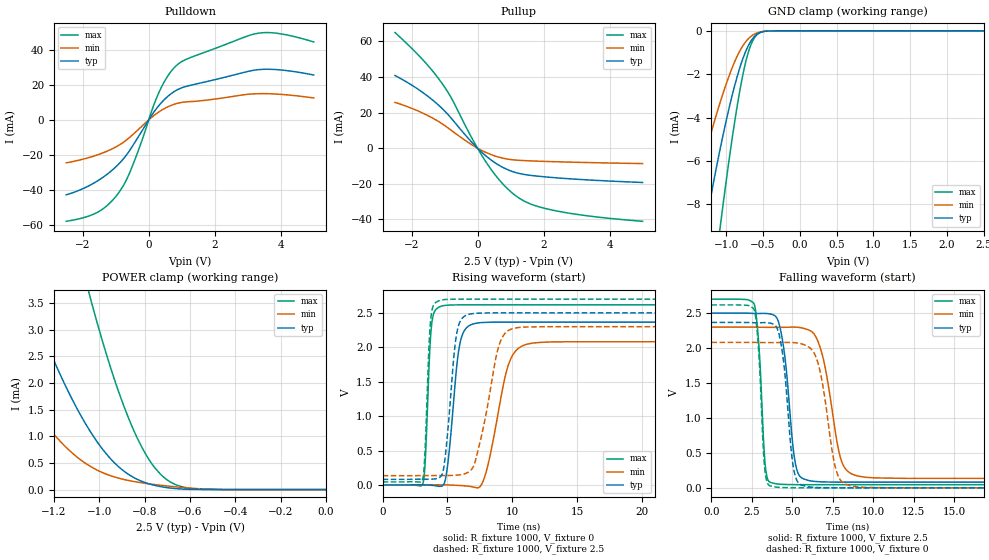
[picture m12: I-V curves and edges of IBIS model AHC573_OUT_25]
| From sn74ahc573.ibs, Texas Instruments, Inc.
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[Model]   AHC573_OUT_25
Model_type  3-state
Enable   Active-Low
Vref =   0.0
Rref =   1000
Cref =   50p
Vmeas =   1.25
| variable   typ   min   max
C_comp   2.25pF   1.96pF   2.41pF
| C_pullup   3.29pF   2.06pF   4.03pF
| C_pulldown   2.98pF   2.14pF   3.95pF
| C_tri-state   2.25pF   1.96pF   2.41pF
[Temperature Range]   40   100   -40
| Ambient temperature   25   85   -40
[Voltage range]   2.5   2.3   2.7
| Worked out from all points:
|   slope of the pulldown table from 0 to 0.375 V, typ, clamps not added: 38.9 ohm
|   slope of the pullup table from 0 to 0.375 V, typ, clamps not added: 61.3 ohm
|   GND clamp passes 1 mA (typ) near -0.74 V on its own axis
|   POWER clamp passes 1 mA (typ) near -1.03 V on its own axis
|   rising waveform, R_fixture 1000, V_fixture 0: 20-80 % time 696ps typ, 1.3ns min, 346ps max; typ from 0 V to 2.37 V
|   falling waveform, R_fixture 1000, V_fixture 2.5: 20-80 % time 597ps typ, 941ps min, 357ps max; typ from 2.5 V to 0.082 V
|   rising waveform, R_fixture 1000, V_fixture 2.5: 20-80 % time 663ps typ, 1.32ns min, 329ps max; typ from 0.082 V to 2.5 V
|   falling waveform, R_fixture 1000, V_fixture 0: 20-80 % time 548ps typ, 827ps min, 337ps max; typ from 2.37 V to 0 V
[GND Clamp]
| AHC573_OUT_25
|   Voltage   I(typ)   I(min)   I(max)
-2.5V     -38.12mA   -24.73mA   -54.32mA
-1.525V   -13.97mA   -8.89mA    -22.06mA
-1.285V   -9.079mA   -5.688mA   -14.78mA
-1.255V   -8.511mA   -5.315mA   -13.91mA
-1.085V   -5.504mA   -3.34mA    -9.154mA
-1.06V    -5.095mA   -3.072mA   -8.49mA
-940mV    -3.279mA   -1.897mA   -5.474mA
-805mV    -1.608mA   -872.9uA   -2.591mA
-710mV    -764.9uA   -407.8uA   -1.124mA
-610mV    -244uA     -144.1uA   -295.3uA
-415mV    -8.6uA     -6.443uA   -5.43uA
2.5V      4.776nA    2.156nA    12.02nA
[POWER Clamp]
| AHC573_OUT_25
|   Voltage   I(typ)   I(min)   I(max)
-2.5V     24.44mA    14.42mA    44.71mA
-1.57V    6.941mA    3.585mA    15.12mA
-1.315V   3.634mA    1.685mA    8.895mA
-1.185V   2.279mA    965.9uA    6.184mA
-1.06V    1.233mA    491.7uA    3.931mA
-1.035V   1.06mA     424.9uA    3.527mA
-935mV    511.3uA    239.6uA    2.092mA
-845mV    219.7uA    150.4uA    1.083mA
-780mV    107uA      108.3uA    559.4uA
-715mV    45.8uA     74.66uA    229.8uA
-585mV    3.146uA    22.88uA    17.46uA
-31.15fV  4.776nA    1.311nA    18.11nA
[Pulldown]
| AHC573_OUT_25
|   Voltage   I(typ)   I(min)   I(max)
-2.5V     -42.7mA    -24.49mA   -57.81mA
-1.54V    -34.65mA   -19.85mA   -52.55mA
-1.21V    -30.24mA   -17.4mA    -47.97mA
-895mV    -24.87mA   -14.36mA   -41.15mA
-495mV    -15.05mA   -8.58mA    -26.34mA
130mV     3.762mA    2.089mA    7.297mA
335mV     8.782mA    4.878mA    16.71mA
630mV     14.23mA    7.881mA    26.48mA
930mV     17.74mA    9.73mA     32.38mA
3.295V    28.59mA    14.93mA    49.33mA
3.97V     28.53mA    14.6mA     49.16mA
5V        25.59mA    12.52mA    44.44mA
[Pullup]
| AHC573_OUT_25
|   Voltage   I(typ)   I(min)   I(max)
-2.5V     40.85mA    25.73mA    64.98mA
-1.72V    32.11mA    20.24mA    50.94mA
-1.15V    23.68mA    14.65mA    38.34mA
-800mV    16.93mA    10.1mA     28.45mA
-175mV    3.382mA    1.944mA    5.825mA
250mV     -4.262mA   -2.344mA   -7.567mA
695mV     -10.06mA   -5.252mA   -18.61mA
1.135V    -13.57mA   -6.625mA   -26.4mA
1.61V     -15.26mA   -7.124mA   -31.38mA
2.33V     -16.56mA   -7.586mA   -35.02mA
3.45V     -17.93mA   -8.108mA   -38.28mA
5V        -19.26mA   -8.64mA    -41.08mA
[Ramp]
| AHC573_OUT_25
| variable   typ   min   max
dV/dt_r   1.43/7.06E-10   1.27/1.32E-09   1.58/3.57E-10
dV/dt_f   1.45/5.98E-10   1.30/9.44E-10   1.59/3.63E-10
R_load = 1000
[Rising Waveform]
| AHC573_OUT_25
R_fixture =   1000
C_fixture =   0
L_fixture =   0
V_fixture =   0
V_fixture_min = 0
V_fixture_max = 0
|   Time   V(typ)   V(min)   V(max)
0s        697.4pV    1.232nV    360.5pV
3.115ns   3.239mV    2.463mV    25.92mV
3.775ns   -4.622mV   3.276mV    2.315V
4.545ns   -18.6mV    2.071mV    2.599V
5.945ns   2.034V     -6.937mV   2.617V
7.015ns   2.341V     -29.59mV   2.617V
7.97ns    2.363V     174.8mV    2.617V
9.78ns    2.366V     1.783V     2.617V
11.16ns   2.366V     2.046V     2.617V
50ns      2.366V     2.081V     2.617V
[Falling Waveform]
| AHC573_OUT_25
R_fixture =   1000
C_fixture =   0
L_fixture =   0
V_fixture =   2.5
V_fixture_min = 2.3
V_fixture_max = 2.7
|   Time   V(typ)   V(min)   V(max)
0s        2.5V       2.3V       2.7V
2.645ns   2.496V     2.3V       2.63V
3.345ns   2.495V     2.297V     282.1mV
3.88ns    2.469V     2.296V     63.5mV
4.465ns   2.002V     2.297V     49.34mV
5.205ns   329mV      2.299V     45.99mV
6ns       105.4mV    2.26V      45.24mV
8.03ns    82.2mV     389.7mV    45.04mV
9.115ns   81.75mV    166mV      45.03mV
50ns      81.66mV    135.1mV    45.03mV
[Rising Waveform]
| AHC573_OUT_25
R_fixture =   1000
C_fixture =   0
L_fixture =   0
V_fixture =   2.5
V_fixture_min = 2.3
V_fixture_max = 2.7
|   Time   V(typ)   V(min)   V(max)
0s        81.66mV    135.1mV    45.03mV
3.07ns    84.73mV    136.9mV    76.09mV
3.71ns    84.4mV     137.3mV    2.4V
4.435ns   114.5mV    136.8mV    2.682V
4.815ns   382.1mV    137.3mV    2.694V
5.715ns   2.195V     142.9mV    2.7V
6.63ns    2.478V     188mV      2.7V
8.98ns    2.5V       2.025V     2.7V
10.1ns    2.5V       2.275V     2.7V
50ns      2.5V       2.3V       2.7V
[Falling Waveform]
| AHC573_OUT_25
R_fixture =   1000
C_fixture =   0
L_fixture =   0
V_fixture =   0
V_fixture_min = 0
V_fixture_max = 0
|   Time   V(typ)   V(min)   V(max)
0s        2.366V     2.081V     2.617V
2.645ns   2.362V     2.081V     2.549V
3.285ns   2.364V     2.078V     302.8mV
3.665ns   2.355V     2.078V     26.4mV
4.345ns   2V         2.079V     4.744mV
5.115ns   232mV      2.077V     996.9uV
5.825ns   22.51mV    2.039V     263uV
7.74ns    527uV      228.2mV    8.375uV
8.65ns    106.5uV    26.99mV    1.734uV
50ns      2.879nV    20.02nV    632pV
